PROGRAM P_Prog1
VAR

	fbKL6401 		: FB_LON_KL6401;

	fbREAD_001		: FB_READ_001_SNVT_amp;
	fbSEND_001		: FB_SEND_001_SNVT_amp;

	fbREAD_002		: FB_READ_002_SNVT_amp_mil;
	fbSEND_002		: FB_SEND_002_SNVT_amp_mil;

	fbREAD_003		: FB_READ_003_SNVT_angle;
	fbSEND_003		: FB_SEND_003_SNVT_angle;

	fbREAD_004		: FB_READ_004_SNVT_angle_vel;
	fbSEND_004		: FB_SEND_004_SNVT_angle_vel;

	fbREAD_005		: FB_READ_005_SNVT_btu_kilo;
	fbSEND_005		: FB_SEND_005_SNVT_btu_kilo;

	fbREAD_006		: FB_READ_006_SNVT_btu_mega;
	fbSEND_006		: FB_SEND_006_SNVT_btu_mega;

	fbREAD_007		: FB_READ_007_SNVT_char_ascii;
	fbSEND_007		: FB_SEND_007_SNVT_char_ascii;

	fbREAD_008		: FB_READ_008_SNVT_count;
	fbSEND_008		: FB_SEND_008_SNVT_count;

	fbREAD_009		: FB_READ_009_SNVT_count_inc;
	fbSEND_009		: FB_SEND_009_SNVT_count_inc;
(*
	fbREAD_010		: FB_READ_011_SNVT_date_day;
	fbSEND_010		: FB_SEND_002_SNVT_amp_mil;
*)

	fbREAD_011		: FB_READ_011_SNVT_date_day;
	fbSEND_011		: FB_SEND_011_SNVT_date_day;

(*
	fbREAD_012		: FB_READ_01;
	fbSEND_012		: FB_SEND_002_SNVT_amp_mil;
*)

	fbREAD_013		: FB_READ_013_SNVT_elec_kwh;
	fbSEND_013		: FB_SEND_013_SNVT_elec_kwh;

	fbREAD_014		: FB_READ_014_SNVT_elec_whr;
	fbSEND_014		: FB_SEND_014_SNVT_elec_whr;

	fbREAD_015		: FB_READ_015_SNVT_flow;
	fbSEND_015		: FB_SEND_015_SNVT_flow;

	fbREAD_016		: FB_READ_016_SNVT_flow_mil;
	fbSEND_016		: FB_SEND_016_SNVT_flow_mil;

	fbREAD_017		: FB_READ_017_SNVT_length;
	fbSEND_017		: FB_SEND_017_SNVT_length;

	fbREAD_018		: FB_READ_018_SNVT_length_kilo;
	fbSEND_018		: FB_SEND_018_SNVT_length_kilo;

	fbREAD_019		: FB_READ_019_SNVT_length_micr;
	fbSEND_019		: FB_SEND_019_SNVT_length_micr;

	fbREAD_020		: FB_READ_020_SNVT_length_mil;
	fbSEND_020		: FB_SEND_020_SNVT_length_mil;

	fbREAD_021		: FB_READ_021_SNVT_lev_cont;
	fbSEND_021		: FB_SEND_021_SNVT_lev_cont;
(*
	fbREAD_022		: FB_READ_022;
	fbSEND_022		: FB_SEND_002_SNVT_amp_mil;
*)
	fbREAD_023		: FB_READ_023_SNVT_mass;
	fbSEND_023		: FB_SEND_023_SNVT_mass;

	fbREAD_024		: FB_READ_024_SNVT_mass_kilo;
	fbSEND_024		: FB_SEND_024_SNVT_mass_kilo;

	fbREAD_025		: FB_READ_025_SNVT_mass_mega;
	fbSEND_025		: FB_SEND_025_SNVT_mass_mega;

	fbREAD_026		: FB_READ_026_SNVT_mass_mil;
	fbSEND_026		: FB_SEND_026_SNVT_mass_mil;

	fbREAD_027		: FB_READ_027_SNVT_power;
	fbSEND_027		: FB_SEND_027_SNVT_power;

	fbREAD_028		: FB_READ_028_SNVT_power_kilo;
	fbSEND_028		: FB_SEND_028_SNVT_power_kilo;

	fbREAD_029		: FB_READ_029_SNVT_ppm;
	fbSEND_029		: FB_SEND_029_SNVT_ppm;

	fbREAD_030		: FB_READ_030_SNVT_press;
	fbSEND_030		: FB_SEND_030_SNVT_press;

	fbREAD_031		: FB_READ_031_SNVT_res;
	fbSEND_031		: FB_SEND_031_SNVT_res;

END_VAR


fbKL6401(
	bDisabled:=FALSE ,
	stParameter_IN:=LON_IN_1 ,
	stParameter_OUT:=LON_OUT_1 ,
	stLON_Com:=stLON_Com_1,
	bReady=> ,
	eError=> ,
	stKL6401=> ,
	arrProgID=> ,
	arrNeuronID=> ,
	bBusy=> ,
	bError=> ,
	dwErrorKL=> ,
	bTimeOut=> ,
	byLONState=> );

(**)
fbREAD_001(
	wNVIndex:=0 ,
	bDisabled:= ,
	stLON_Com:=stLON_Com_1,
	rValue=> ,
	bNewData=> ,
	bError=> ,
	eError=> );
fbREAD_001.rValue;
fbREAD_001.bError;
fbREAD_001.eError;

fbSEND_001.rValue;
fbSEND_001.bStart;
fbSEND_001.bError;
fbSEND_001.eError;
fbSEND_001.bBusy;
fbSEND_001.dwErrorKL;

fbSEND_001.bAuto;
fbSEND_001.bSendInit;
fbSEND_001.tMinSendTime;
fbSEND_001.tMaxSendTime;
fbSEND_001.rValueLimit;

fbSEND_001(
	wNVIndex:=1 ,
	bStart:= ,
	rValue:= ,
	bDisabled:= ,
	stLON_Com:=stLON_Com_1,
	bError=> ,
	eError=> );
fbSEND_001.bStart:=FALSE;

(**)
fbREAD_002(
	wNVIndex:=2 ,
	bDisabled:= ,
	stLON_Com:=stLON_Com_1,
	rValue=> ,
	bNewData=> ,
	bError=> ,
	eError=> );
fbREAD_002.rValue;
fbREAD_002.bError;
fbREAD_002.eError;

fbSEND_002.rValue;
fbSEND_002.bStart;
fbSEND_002.bError;
fbSEND_002.eError;
fbSEND_002.bBusy;
fbSEND_002.dwErrorKL;

fbSEND_002.bAuto;
fbSEND_002.bSendInit;
fbSEND_002.tMinSendTime;
fbSEND_002.tMaxSendTime;
fbSEND_002.rValueLimit;

fbSEND_002(
	wNVIndex:=3 ,
	bStart:= ,
	rValue:= ,
	bDisabled:= ,
	stLON_Com:=stLON_Com_1,
	bError=> ,
	eError=> );
fbSEND_002.bStart:=FALSE;

(**)
fbREAD_003(
	wNVIndex:=4 ,
	bDisabled:= ,
	stLON_Com:=stLON_Com_1,
	rValue=> ,
	bNewData=> ,
	bError=> ,
	eError=> );
fbREAD_003.rValue;
fbREAD_003.bError;
fbREAD_003.eError;
fbSEND_003.bBusy;
fbSEND_003.dwErrorKL;

fbSEND_003.rValue;
fbSEND_003.bStart;
fbSEND_003.bError;
fbSEND_003.eError;

fbSEND_003.bAuto;
fbSEND_003.bSendInit;
fbSEND_003.tMinSendTime;
fbSEND_003.tMaxSendTime;
fbSEND_003.rValueLimit;

fbSEND_003(
	wNVIndex:=5 ,
	bStart:= ,
	rValue:= ,
	bDisabled:= ,
	stLON_Com:=stLON_Com_1,
	bError=> ,
	eError=> );
fbSEND_003.bStart:=FALSE;

(**)
fbREAD_004(
	wNVIndex:=6 ,
	bDisabled:= ,
	stLON_Com:=stLON_Com_1,
	rValue=> ,
	bNewData=> ,
	bError=> ,
	eError=> );
fbREAD_004.rValue;
fbREAD_004.bError;
fbREAD_004.eError;

fbSEND_004.rValue;
fbSEND_004.bStart;
fbSEND_004.bError;
fbSEND_004.eError;
fbSEND_004.bBusy;
fbSEND_004.dwErrorKL;

fbSEND_004.bAuto;
fbSEND_004.bSendInit;
fbSEND_004.tMinSendTime;
fbSEND_004.tMaxSendTime;
fbSEND_004.rValueLimit;

fbSEND_004(
	wNVIndex:=7 ,
	bStart:= ,
	rValue:= ,
	bDisabled:= ,
	stLON_Com:=stLON_Com_1,
	bError=> ,
	eError=> );
fbSEND_004.bStart:=FALSE;

(**)
fbREAD_005(
	wNVIndex:=8 ,
	bDisabled:= ,
	stLON_Com:=stLON_Com_1,
	uiValue=> ,
	bNewData=> ,
	bError=> ,
	eError=> );
fbREAD_005.uiValue;
fbREAD_005.bError;
fbREAD_005.eError;
fbSEND_005.bBusy;
fbSEND_005.dwErrorKL;

fbSEND_005.uiValue;
fbSEND_005.bStart;
fbSEND_005.bError;
fbSEND_005.eError;
fbSEND_005.bBusy;
fbSEND_005.dwErrorKL;

fbSEND_005.bAuto;
fbSEND_005.bSendInit;
fbSEND_005.tMinSendTime;
fbSEND_005.tMaxSendTime;
fbSEND_005.uiValueLimit;

fbSEND_005(
	wNVIndex:=9 ,
	bStart:= ,
	uiValue:= ,
	bDisabled:= ,
	stLON_Com:=stLON_Com_1,
	bError=> ,
	eError=> );
fbSEND_005.bStart:=FALSE;

(**)
fbREAD_006(
	wNVIndex:=10 ,
	bDisabled:= ,
	stLON_Com:=stLON_Com_1,
	uiValue=> ,
	bNewData=> ,
	bError=> ,
	eError=> );
fbREAD_006.uiValue;
fbREAD_006.bError;
fbREAD_006.eError;

fbSEND_006.uiValue;
fbSEND_006.bStart;
fbSEND_006.bError;
fbSEND_006.eError;
fbSEND_006.bBusy;
fbSEND_006.dwErrorKL;

fbSEND_006.bAuto;
fbSEND_006.bSendInit;
fbSEND_006.tMinSendTime;
fbSEND_006.tMaxSendTime;
fbSEND_006.uiValueLimit;

fbSEND_006(
	wNVIndex:=11 ,
	bStart:= ,
	uiValue:= ,
	bDisabled:= ,
	stLON_Com:=stLON_Com_1,
	bError=> ,
	eError=> );
fbSEND_006.bStart:=FALSE;

(**)
fbREAD_007(
	wNVIndex:=12 ,
	bDisabled:= ,
	stLON_Com:=stLON_Com_1,
	sValue=> ,
	bNewData=> ,
	bError=> ,
	eError=> );
fbREAD_007.sValue;
fbREAD_007.bError;
fbREAD_007.eError;

fbSEND_007.sValue;
fbSEND_007.bStart;
fbSEND_007.bError;
fbSEND_007.eError;
fbSEND_007.bBusy;
fbSEND_007.dwErrorKL;

fbSEND_007.bAuto;
fbSEND_007.bSendInit;
fbSEND_007.tMinSendTime;
fbSEND_007.tMaxSendTime;
(*fbSEND_007.rValueLimit;*)

fbSEND_007(
	wNVIndex:=13 ,
	bStart:= ,
	sValue:= ,
	bDisabled:= ,
	stLON_Com:=stLON_Com_1,
	bError=> ,
	eError=> );
fbSEND_007.bStart:=FALSE;

(**)
fbREAD_008(
	wNVIndex:=14 ,
	bDisabled:= ,
	stLON_Com:=stLON_Com_1,
	uiValue=> ,
	bNewData=> ,
	bError=> ,
	eError=> );
fbREAD_008.uiValue;
fbREAD_008.bError;
fbREAD_008.eError;

fbSEND_008.uiValue;
fbSEND_008.bStart;
fbSEND_008.bError;
fbSEND_008.eError;
fbSEND_008.bBusy;
fbSEND_008.dwErrorKL;

fbSEND_008.bAuto;
fbSEND_008.bSendInit;
fbSEND_008.tMinSendTime;
fbSEND_008.tMaxSendTime;
fbSEND_008.uiValue;

fbSEND_008(
	wNVIndex:=15 ,
	bStart:= ,
	uiValue:= ,
	bDisabled:= ,
	stLON_Com:=stLON_Com_1,
	bError=> ,
	eError=> );
fbSEND_008.bStart:=FALSE;

(**)
fbREAD_009(
	wNVIndex:=16 ,
	bDisabled:= ,
	stLON_Com:=stLON_Com_1,
	iValue=> ,
	bNewData=> ,
	bError=> ,
	eError=> );
fbREAD_009.iValue;
fbREAD_009.bError;
fbREAD_009.eError;

fbSEND_009.iValue;
fbSEND_009.bStart;
fbSEND_009.bError;
fbSEND_009.eError;
fbSEND_009.bBusy;
fbSEND_009.dwErrorKL;

fbSEND_009.bAuto;
fbSEND_009.bSendInit;
fbSEND_009.tMinSendTime;
fbSEND_009.tMaxSendTime;
fbSEND_009.iValueLimit;

fbSEND_009(
	wNVIndex:=17 ,
	bStart:= ,
	iValue:= ,
	bDisabled:= ,
	stLON_Com:=stLON_Com_1,
	bError=> ,
	eError=> );
fbSEND_009.bStart:=FALSE;

(*10*)

(**)
fbREAD_011(
	wNVIndex:=20 ,
	bDisabled:= ,
	stLON_Com:=stLON_Com_1,
	eValue=> ,
	bNewData=> ,
	bError=> ,
	eError=> );
fbREAD_011.eValue;
fbREAD_011.bError;
fbREAD_011.eError;

fbSEND_011.eValue;
fbSEND_011.bStart;
fbSEND_011.bError;
fbSEND_011.eError;
fbSEND_011.bBusy;
fbSEND_011.dwErrorKL;

fbSEND_011.bAuto;
fbSEND_011.bSendInit;
fbSEND_011.tMinSendTime;
fbSEND_011.tMaxSendTime;

fbSEND_011(
	wNVIndex:=21 ,
	bStart:= ,
	eValue:= ,
	bDisabled:= ,
	stLON_Com:=stLON_Com_1,
	bError=> ,
	eError=> );
fbSEND_011.bStart:=FALSE;

(*12*)

(**)
fbREAD_013(
	wNVIndex:=24 ,
	bDisabled:= ,
	stLON_Com:=stLON_Com_1,
	uiValue=> ,
	bNewData=> ,
	bError=> ,
	eError=> );
fbREAD_013.uiValue;
fbREAD_013.bError;
fbREAD_013.eError;

fbSEND_013.uiValue;
fbSEND_013.bStart;
fbSEND_013.bError;
fbSEND_013.eError;
fbSEND_013.bBusy;
fbSEND_013.dwErrorKL;

fbSEND_013.bAuto;
fbSEND_013.bSendInit;
fbSEND_013.tMinSendTime;
fbSEND_013.tMaxSendTime;
fbSEND_013.uiValueLimit;

fbSEND_013(
	wNVIndex:=25 ,
	bStart:= ,
	uiValue:= ,
	bDisabled:= ,
	stLON_Com:=stLON_Com_1,
	bError=> ,
	eError=> );
fbSEND_013.bStart:=FALSE;

(**)
fbREAD_014(
	wNVIndex:=26 ,
	bDisabled:= ,
	stLON_Com:=stLON_Com_1,
	rValue=> ,
	bNewData=> ,
	bError=> ,
	eError=> );
fbREAD_014.rValue;
fbREAD_014.bError;
fbREAD_014.eError;

fbSEND_014.rValue;
fbSEND_014.bStart;
fbSEND_014.bError;
fbSEND_014.eError;
fbSEND_014.bBusy;
fbSEND_014.dwErrorKL;

fbSEND_014.bAuto;
fbSEND_014.bSendInit;
fbSEND_014.tMinSendTime;
fbSEND_014.tMaxSendTime;
fbSEND_014.rValueLimit;

fbSEND_014(
	wNVIndex:=27 ,
	bStart:= ,
	rValue:= ,
	bDisabled:= ,
	stLON_Com:=stLON_Com_1,
	bError=> ,
	eError=> );
fbSEND_014.bStart:=FALSE;

(**)
fbREAD_015(
	wNVIndex:=28 ,
	bDisabled:= ,
	stLON_Com:=stLON_Com_1,
	uiValue=> ,
	bNewData=> ,
	bError=> ,
	eError=> );
fbREAD_015.uiValue;
fbREAD_015.bError;
fbREAD_015.eError;

fbSEND_015.uiValue;
fbSEND_015.bStart;
fbSEND_015.bError;
fbSEND_015.eError;
fbSEND_015.bBusy;
fbSEND_015.dwErrorKL;

fbSEND_015.bAuto;
fbSEND_015.bSendInit;
fbSEND_015.tMinSendTime;
fbSEND_015.tMaxSendTime;
fbSEND_015.uiValueLimit;

fbSEND_015(
	wNVIndex:=29 ,
	bStart:= ,
	uiValue:= ,
	bDisabled:= ,
	stLON_Com:=stLON_Com_1,
	bError=> ,
	eError=> );
fbSEND_015.bStart:=FALSE;


(**)
fbREAD_016(
	wNVIndex:=30 ,
	bDisabled:= ,
	stLON_Com:=stLON_Com_1,
	uiValue=> ,
	bNewData=> ,
	bError=> ,
	eError=> );
fbREAD_016.uiValue;
fbREAD_016.bError;
fbREAD_016.eError;

fbSEND_016.uiValue;
fbSEND_016.bStart;
fbSEND_016.bError;
fbSEND_016.eError;
fbSEND_016.bBusy;
fbSEND_016.dwErrorKL;

fbSEND_016.bAuto;
fbSEND_016.bSendInit;
fbSEND_016.tMinSendTime;
fbSEND_016.tMaxSendTime;
fbSEND_016.uiValueLimit;

fbSEND_016(
	wNVIndex:=31 ,
	bStart:= ,
	uiValue:= ,
	bDisabled:= ,
	stLON_Com:=stLON_Com_1,
	bError=> ,
	eError=> );
fbSEND_016.bStart:=FALSE;

(**)
fbREAD_017(
	wNVIndex:=32 ,
	bDisabled:= ,
	stLON_Com:=stLON_Com_1,
	rValue=> ,
	bNewData=> ,
	bError=> ,
	eError=> );
fbREAD_017.rValue;
fbREAD_017.bError;
fbREAD_017.eError;

fbSEND_017.rValue;
fbSEND_017.bStart;
fbSEND_017.bError;
fbSEND_017.eError;
fbSEND_017.bBusy;
fbSEND_017.dwErrorKL;

fbSEND_017.bAuto;
fbSEND_017.bSendInit;
fbSEND_017.tMinSendTime;
fbSEND_017.tMaxSendTime;
fbSEND_017.rValueLimit;

fbSEND_017(
	wNVIndex:=33 ,
	bStart:= ,
	rValue:= ,
	bDisabled:= ,
	stLON_Com:=stLON_Com_1,
	bError=> ,
	eError=> );
fbSEND_017.bStart:=FALSE;

(**)
fbREAD_018(
	wNVIndex:=34 ,
	bDisabled:= ,
	stLON_Com:=stLON_Com_1,
	rValue=> ,
	bNewData=> ,
	bError=> ,
	eError=> );
fbREAD_018.rValue;
fbREAD_018.bError;
fbREAD_018.eError;

fbSEND_018.rValue;
fbSEND_018.bStart;
fbSEND_018.bError;
fbSEND_018.eError;
fbSEND_018.bBusy;
fbSEND_018.dwErrorKL;

fbSEND_018.bAuto;
fbSEND_018.bSendInit;
fbSEND_018.tMinSendTime;
fbSEND_018.tMaxSendTime;
fbSEND_018.rValueLimit;

fbSEND_018(
	wNVIndex:=35 ,
	bStart:= ,
	rValue:= ,
	bDisabled:= ,
	stLON_Com:=stLON_Com_1,
	bError=> ,
	eError=> );
fbSEND_018.bStart:=FALSE;

(**)
fbREAD_019(
	wNVIndex:=36 ,
	bDisabled:= ,
	stLON_Com:=stLON_Com_1,
	rValue=> ,
	bNewData=> ,
	bError=> ,
	eError=> );
fbREAD_019.rValue;
fbREAD_019.bError;
fbREAD_019.eError;

fbSEND_019.rValue;
fbSEND_019.bStart;
fbSEND_019.bError;
fbSEND_019.eError;
fbSEND_019.bBusy;
fbSEND_019.dwErrorKL;

fbSEND_019.bAuto;
fbSEND_019.bSendInit;
fbSEND_019.tMinSendTime;
fbSEND_019.tMaxSendTime;
fbSEND_019.rValueLimit;

fbSEND_019(
	wNVIndex:=37 ,
	bStart:= ,
	rValue:= ,
	bDisabled:= ,
	stLON_Com:=stLON_Com_1,
	bError=> ,
	eError=> );
fbSEND_019.bStart:=FALSE;

(**)
fbREAD_020(
	wNVIndex:=38 ,
	bDisabled:= ,
	stLON_Com:=stLON_Com_1,
	rValue=> ,
	bNewData=> ,
	bError=> ,
	eError=> );
fbREAD_020.rValue;
fbREAD_020.bError;
fbREAD_020.eError;

fbSEND_020.rValue;
fbSEND_020.bStart;
fbSEND_020.bError;
fbSEND_020.eError;
fbSEND_020.bBusy;
fbSEND_020.dwErrorKL;

fbSEND_020.bAuto;
fbSEND_020.bSendInit;
fbSEND_020.tMinSendTime;
fbSEND_020.tMaxSendTime;
fbSEND_020.rValueLimit;

fbSEND_020(
	wNVIndex:=39 ,
	bStart:= ,
	rValue:= ,
	bDisabled:= ,
	stLON_Com:=stLON_Com_1,
	bError=> ,
	eError=> );
fbSEND_020.bStart:=FALSE;

(**)
fbREAD_021(
	wNVIndex:=40 ,
	bDisabled:= ,
	stLON_Com:=stLON_Com_1,
	rValue=> ,
	bNewData=> ,
	bError=> ,
	eError=> );
fbREAD_021.rValue;
fbREAD_021.bError;
fbREAD_021.eError;

fbSEND_021.rValue;
fbSEND_021.bStart;
fbSEND_021.bError;
fbSEND_021.eError;
fbSEND_021.bBusy;
fbSEND_021.dwErrorKL;

fbSEND_021.bAuto;
fbSEND_021.bSendInit;
fbSEND_021.tMinSendTime;
fbSEND_021.tMaxSendTime;
fbSEND_021.rValueLimit;

fbSEND_021(
	wNVIndex:=41 ,
	bStart:= ,
	rValue:= ,
	bDisabled:= ,
	stLON_Com:=stLON_Com_1,
	bError=> ,
	eError=> );
fbSEND_021.bStart:=FALSE;

(*22*)

(**)
fbREAD_023(
	wNVIndex:=44 ,
	bDisabled:= ,
	stLON_Com:=stLON_Com_1,
	rValue=> ,
	bNewData=> ,
	bError=> ,
	eError=> );
fbREAD_023.rValue;
fbREAD_023.bError;
fbREAD_023.eError;

fbSEND_023.rValue;
fbSEND_023.bStart;
fbSEND_023.bError;
fbSEND_023.eError;
fbSEND_023.bBusy;
fbSEND_023.dwErrorKL;

fbSEND_023.bAuto;
fbSEND_023.bSendInit;
fbSEND_023.tMinSendTime;
fbSEND_023.tMaxSendTime;
fbSEND_023.rValueLimit;

fbSEND_023(
	wNVIndex:=45 ,
	bStart:= ,
	rValue:= ,
	bDisabled:= ,
	stLON_Com:=stLON_Com_1,
	bError=> ,
	eError=> );
fbSEND_023.bStart:=FALSE;

(**)
fbREAD_024(
	wNVIndex:=46 ,
	bDisabled:= ,
	stLON_Com:=stLON_Com_1,
	rValue=> ,
	bNewData=> ,
	bError=> ,
	eError=> );
fbREAD_024.rValue;
fbREAD_024.bError;
fbREAD_024.eError;

fbSEND_024.rValue;
fbSEND_024.bStart;
fbSEND_024.bError;
fbSEND_024.eError;
fbSEND_024.bBusy;
fbSEND_024.dwErrorKL;

fbSEND_024.bAuto;
fbSEND_024.bSendInit;
fbSEND_024.tMinSendTime;
fbSEND_024.tMaxSendTime;
fbSEND_024.rValueLimit;

fbSEND_024(
	wNVIndex:=47 ,
	bStart:= ,
	rValue:= ,
	bDisabled:= ,
	stLON_Com:=stLON_Com_1,
	bError=> ,
	eError=> );
fbSEND_024.bStart:=FALSE;

(**)
fbREAD_025(
	wNVIndex:=48 ,
	bDisabled:= ,
	stLON_Com:=stLON_Com_1,
	rValue=> ,
	bNewData=> ,
	bError=> ,
	eError=> );
fbREAD_025.rValue;
fbREAD_025.bError;
fbREAD_025.eError;

fbSEND_025.rValue;
fbSEND_025.bStart;
fbSEND_025.bError;
fbSEND_025.eError;
fbSEND_025.bBusy;
fbSEND_025.dwErrorKL;

fbSEND_025.bAuto;
fbSEND_025.bSendInit;
fbSEND_025.tMinSendTime;
fbSEND_025.tMaxSendTime;
fbSEND_025.rValueLimit;

fbSEND_025(
	wNVIndex:=49 ,
	bStart:= ,
	rValue:= ,
	bDisabled:= ,
	stLON_Com:=stLON_Com_1,
	bError=> ,
	eError=> );
fbSEND_025.bStart:=FALSE;

(**)
fbREAD_026(
	wNVIndex:=50 ,
	bDisabled:= ,
	stLON_Com:=stLON_Com_1,
	rValue=> ,
	bNewData=> ,
	bError=> ,
	eError=> );
fbREAD_026.rValue;
fbREAD_026.bError;
fbREAD_026.eError;

fbSEND_026.rValue;
fbSEND_026.bStart;
fbSEND_026.bError;
fbSEND_026.eError;
fbSEND_026.bBusy;
fbSEND_026.dwErrorKL;

fbSEND_026.bAuto;
fbSEND_026.bSendInit;
fbSEND_026.tMinSendTime;
fbSEND_026.tMaxSendTime;
fbSEND_026.rValueLimit;

fbSEND_026(
	wNVIndex:=51 ,
	bStart:= ,
	rValue:= ,
	bDisabled:= ,
	stLON_Com:=stLON_Com_1,
	bError=> ,
	eError=> );
fbSEND_026.bStart:=FALSE;

(**)
fbREAD_027(
	wNVIndex:=52 ,
	bDisabled:= ,
	stLON_Com:=stLON_Com_1,
	rValue=> ,
	bNewData=> ,
	bError=> ,
	eError=> );
fbREAD_027.rValue;
fbREAD_027.bError;
fbREAD_027.eError;

fbSEND_027.rValue;
fbSEND_027.bStart;
fbSEND_027.bError;
fbSEND_027.eError;
fbSEND_027.bBusy;
fbSEND_027.dwErrorKL;

fbSEND_027.bAuto;
fbSEND_027.bSendInit;
fbSEND_027.tMinSendTime;
fbSEND_027.tMaxSendTime;
fbSEND_027.rValueLimit;

fbSEND_027(
	wNVIndex:=53 ,
	bStart:= ,
	rValue:= ,
	bDisabled:= ,
	stLON_Com:=stLON_Com_1,
	bError=> ,
	eError=> );
fbSEND_027.bStart:=FALSE;

(**)
fbREAD_028(
	wNVIndex:=54 ,
	bDisabled:= ,
	stLON_Com:=stLON_Com_1,
	rValue=> ,
	bNewData=> ,
	bError=> ,
	eError=> );
fbREAD_028.rValue;
fbREAD_028.bError;
fbREAD_028.eError;

fbSEND_028.rValue;
fbSEND_028.bStart;
fbSEND_028.bError;
fbSEND_028.eError;
fbSEND_028.bBusy;
fbSEND_028.dwErrorKL;

fbSEND_028.bAuto;
fbSEND_028.bSendInit;
fbSEND_028.tMinSendTime;
fbSEND_028.tMaxSendTime;
fbSEND_028.rValueLimit;

fbSEND_028(
	wNVIndex:=55 ,
	bStart:= ,
	rValue:= ,
	bDisabled:= ,
	stLON_Com:=stLON_Com_1,
	bError=> ,
	eError=> );
fbSEND_028.bStart:=FALSE;

(**)
fbREAD_029(
	wNVIndex:=56 ,
	bDisabled:= ,
	stLON_Com:=stLON_Com_1,
	uiValue=> ,
	bNewData=> ,
	bError=> ,
	eError=> );
fbREAD_029.uiValue;
fbREAD_029.bError;
fbREAD_029.eError;

fbSEND_029.uiValue;
fbSEND_029.bStart;
fbSEND_029.bError;
fbSEND_029.eError;
fbSEND_029.bBusy;
fbSEND_029.dwErrorKL;

fbSEND_029.bAuto;
fbSEND_029.bSendInit;
fbSEND_029.tMinSendTime;
fbSEND_029.tMaxSendTime;
fbSEND_029.uiValueLimit;

fbSEND_029(
	wNVIndex:=57 ,
	bStart:= ,
	uiValue:= ,
	bDisabled:= ,
	stLON_Com:=stLON_Com_1,
	bError=> ,
	eError=> );
fbSEND_029.bStart:=FALSE;

(**)
fbREAD_030(
	wNVIndex:=58 ,
	bDisabled:= ,
	stLON_Com:=stLON_Com_1,
	rValue=> ,
	bNewData=> ,
	bError=> ,
	eError=> );
fbREAD_030.rValue;
fbREAD_030.bError;
fbREAD_030.eError;

fbSEND_030.rValue;
fbSEND_030.bStart;
fbSEND_030.bError;
fbSEND_030.eError;
fbSEND_030.bBusy;
fbSEND_030.dwErrorKL;

fbSEND_030.bAuto;
fbSEND_030.bSendInit;
fbSEND_030.tMinSendTime;
fbSEND_030.tMaxSendTime;
fbSEND_030.rValueLimit;

fbSEND_030(
	wNVIndex:=59 ,
	bStart:= ,
	rValue:= ,
	bDisabled:= ,
	stLON_Com:=stLON_Com_1,
	bError=> ,
	eError=> );
fbSEND_030.bStart:=FALSE;


(**)
fbREAD_031(
	wNVIndex:=60 ,
	bDisabled:= ,
	stLON_Com:=stLON_Com_1,
	rValue=> ,
	bNewData=> ,
	bError=> ,
	eError=> );
fbREAD_031.rValue;
fbREAD_031.bError;
fbREAD_031.eError;

fbSEND_031.rValue;
fbSEND_031.bStart;
fbSEND_031.bError;
fbSEND_031.eError;
fbSEND_031.bBusy;
fbSEND_031.dwErrorKL;

fbSEND_031.bAuto;
fbSEND_031.bSendInit;
fbSEND_031.tMinSendTime;
fbSEND_031.tMaxSendTime;
fbSEND_031.rValueLimit;

fbSEND_031(
	wNVIndex:=61 ,
	bStart:= ,
	rValue:= ,
	bDisabled:= ,
	stLON_Com:=stLON_Com_1,
	bError=> ,
	eError=> );
fbSEND_031.bStart:=FALSE;

END_PROGRAM
